(* Logix 5000 AddOnInstructionDefinition export Banner_Q5X_5000_Param_v4; software revision 33.00; part 3 of 3 *)
(* tags used below, declared in another part *)
   Q5X : Banner_Q5X_5000_v4;
   Port_Data : Banner_IOL_Port_v4;
   Port : DINT;
   Local_Control : DINT;
   Command_Being_Processed : BOOL;
   Update_Archive : BOOL;
   Index_Write_Inprocess : INT;
   Inprocess_Index : DINT;
(* Banner_Q5X_5000_Param_v4, continued *)

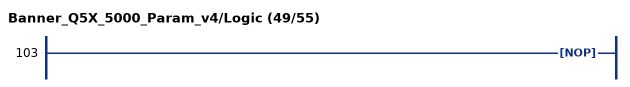
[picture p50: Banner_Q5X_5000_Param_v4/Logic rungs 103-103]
   103: NOP();
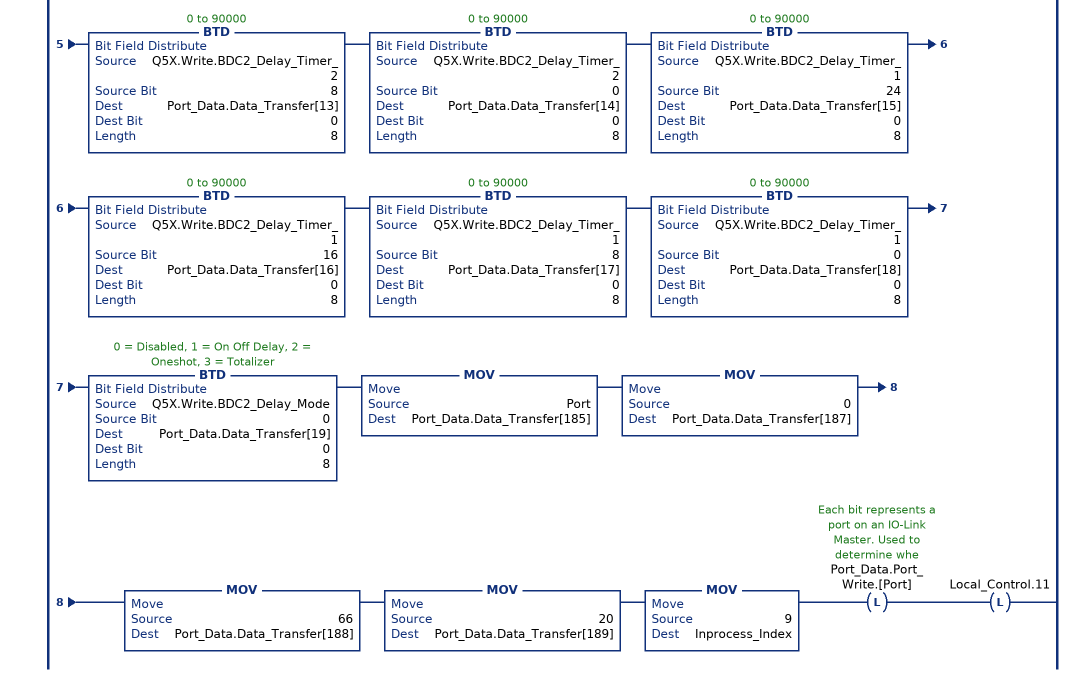
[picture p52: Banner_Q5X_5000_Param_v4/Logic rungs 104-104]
   // ************************************************************************************************************
   // Section of AOI that controls writing of the BDC2 Vendor Specific Configuration parameter (index 66).
   // ************************************************************************************************************
   104: XIC(Q5X.Initial_Global_Read)XIO(Command_Being_Processed)XIO(Local_Control.11)EQU(Q5X.Command,51)OTL(Command_Being_Processed)BTD(Q5X.Write.BDC2_Auto_Thresholding,0,Port_Data.Data_Transfer[0],0,8)BTD(Q5X.Write.BDC2_User_FGS_Window_Size,24,Port_Data.Data_Transfer[1],0,8)BTD(Q5X.Write.BDC2_User_FGS_Window_Size,16,Port_Data.Data_Transfer[2],0,8)BTD(Q5X.Write.BDC2_User_FGS_Window_Size,8,Port_Data.Data_Transfer[3],0,8)BTD(Q5X.Write.BDC2_User_FGS_Window_Size,0,Port_Data.Data_Transfer[4],0,8)BTD(Q5X.Write.BDC2_User_Teach_Offset,24,Port_Data.Data_Transfer[5],0,8)BTD(Q5X.Write.BDC2_User_Teach_Offset,16,Port_Data.Data_Transfer[6],0,8)BTD(Q5X.Write.BDC2_User_Teach_Offset,8,Port_Data.Data_Transfer[7],0,8)BTD(Q5X.Write.BDC2_User_Teach_Offset,0,Port_Data.Data_Transfer[8],0,8)BTD(Q5X.Write.BDC2_FGS_Window_Size,0,Port_Data.Data_Transfer[9],0,8)BTD(Q5X.Write.BDC2_BGS_Teach_Offset,0,Port_Data.Data_Transfer[10],0,8)BTD(Q5X.Write.BDC2_Delay_Timer_2,24,Port_Data.Data_Transfer[11],0,8)BTD(Q5X.Write.BDC2_Delay_Timer_2,16,Port_Data.Data_Transfer[12],0,8)BTD(Q5X.Write.BDC2_Delay_Timer_2,8,Port_Data.Data_Transfer[13],0,8)BTD(Q5X.Write.BDC2_Delay_Timer_2,0,Port_Data.Data_Transfer[14],0,8)BTD(Q5X.Write.BDC2_Delay_Timer_1,24,Port_Data.Data_Transfer[15],0,8)BTD(Q5X.Write.BDC2_Delay_Timer_1,16,Port_Data.Data_Transfer[16],0,8)BTD(Q5X.Write.BDC2_Delay_Timer_1,8,Port_Data.Data_Transfer[17],0,8)BTD(Q5X.Write.BDC2_Delay_Timer_1,0,Port_Data.Data_Transfer[18],0,8)BTD(Q5X.Write.BDC2_Delay_Mode,0,Port_Data.Data_Transfer[19],0,8)MOV(Port,Port_Data.Data_Transfer[185])MOV(0,Port_Data.Data_Transfer[187])MOV(66,Port_Data.Data_Transfer[188])MOV(20,Port_Data.Data_Transfer[189])MOV(9,Inprocess_Index)OTL(Port_Data.Port_Write.[Port])OTL(Local_Control.11);
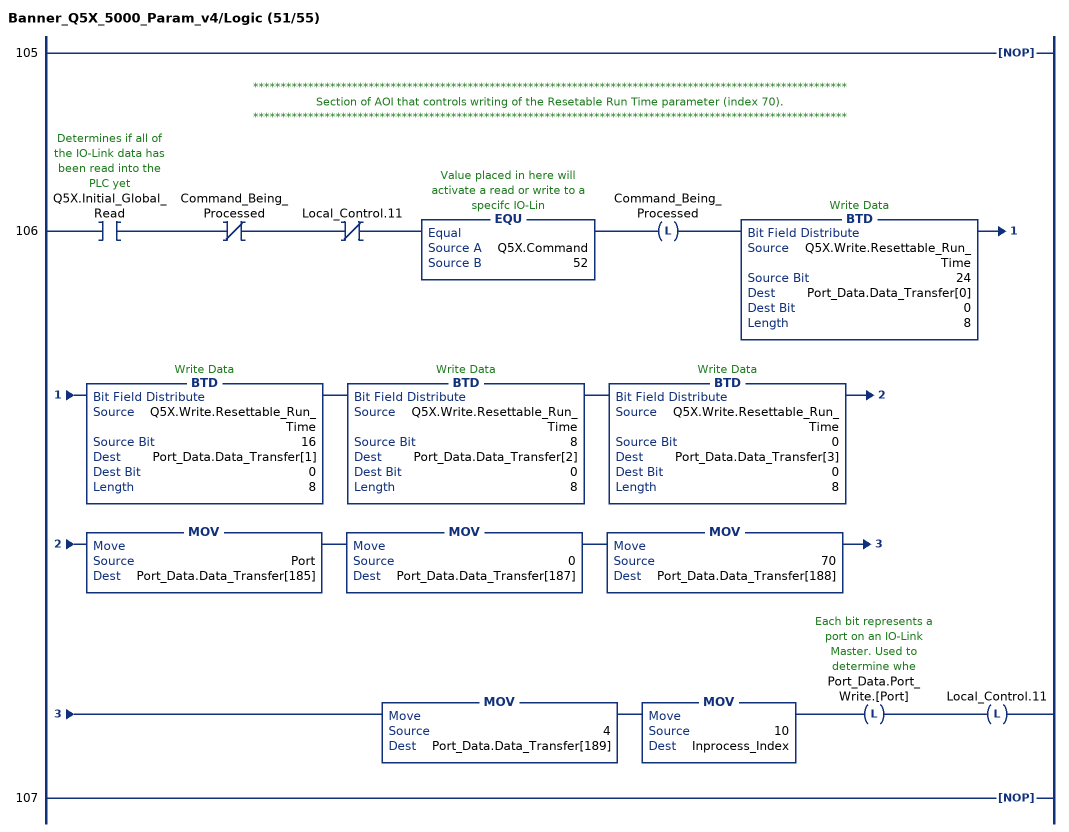
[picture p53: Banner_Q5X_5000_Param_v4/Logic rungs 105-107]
   105: NOP();
   // ************************************************************************************************************
   // Section of AOI that controls writing of the Resetable Run Time parameter (index 70).
   // ************************************************************************************************************
   106: XIC(Q5X.Initial_Global_Read)XIO(Command_Being_Processed)XIO(Local_Control.11)EQU(Q5X.Command,52)OTL(Command_Being_Processed)BTD(Q5X.Write.Resettable_Run_Time,24,Port_Data.Data_Transfer[0],0,8)BTD(Q5X.Write.Resettable_Run_Time,16,Port_Data.Data_Transfer[1],0,8)BTD(Q5X.Write.Resettable_Run_Time,8,Port_Data.Data_Transfer[2],0,8)BTD(Q5X.Write.Resettable_Run_Time,0,Port_Data.Data_Transfer[3],0,8)MOV(Port,Port_Data.Data_Transfer[185])MOV(0,Port_Data.Data_Transfer[187])MOV(70,Port_Data.Data_Transfer[188])MOV(4,Port_Data.Data_Transfer[189])MOV(10,Inprocess_Index)OTL(Port_Data.Port_Write.[Port])OTL(Local_Control.11);
   107: NOP();
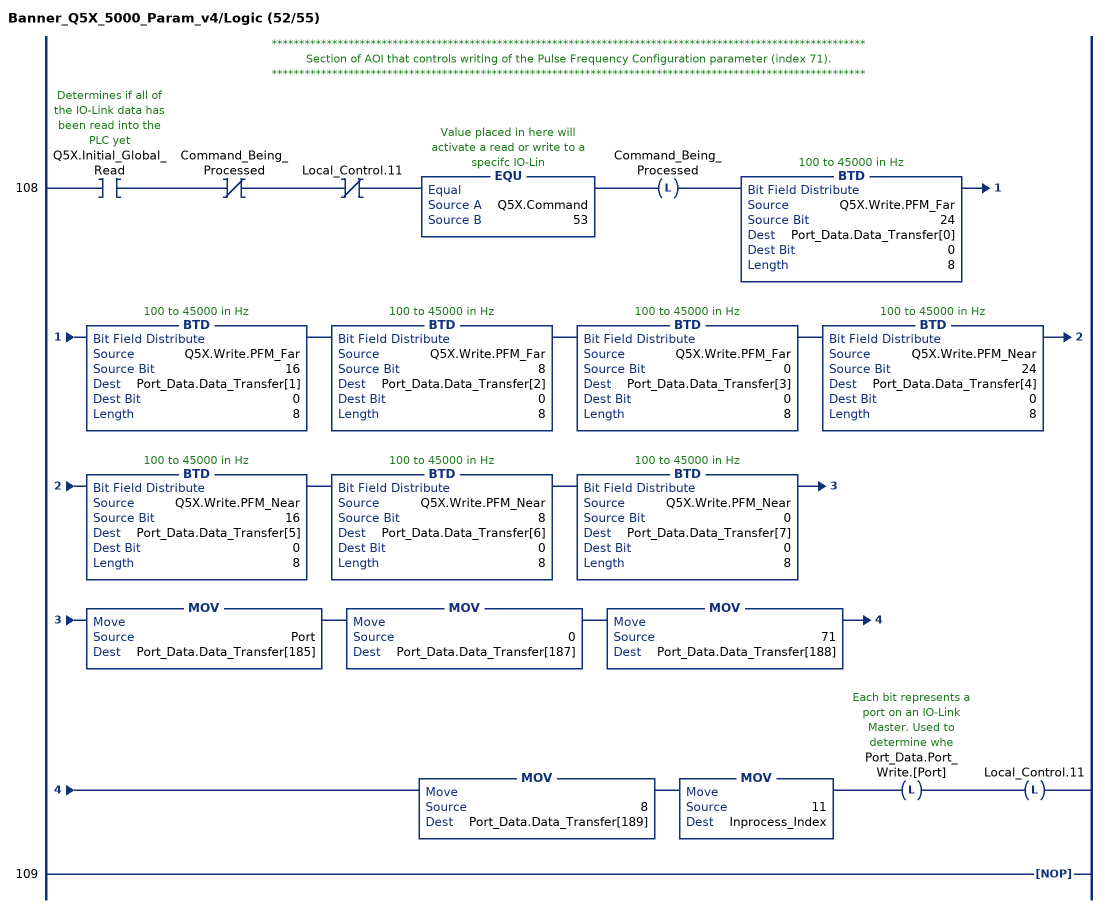
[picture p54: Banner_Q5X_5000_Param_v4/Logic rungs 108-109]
   // ************************************************************************************************************
   // Section of AOI that controls writing of the Pulse Frequency Configuration parameter (index 71).
   // ************************************************************************************************************
   108: XIC(Q5X.Initial_Global_Read)XIO(Command_Being_Processed)XIO(Local_Control.11)EQU(Q5X.Command,53)OTL(Command_Being_Processed)BTD(Q5X.Write.PFM_Far,24,Port_Data.Data_Transfer[0],0,8)BTD(Q5X.Write.PFM_Far,16,Port_Data.Data_Transfer[1],0,8)BTD(Q5X.Write.PFM_Far,8,Port_Data.Data_Transfer[2],0,8)BTD(Q5X.Write.PFM_Far,0,Port_Data.Data_Transfer[3],0,8)BTD(Q5X.Write.PFM_Near,24,Port_Data.Data_Transfer[4],0,8)BTD(Q5X.Write.PFM_Near,16,Port_Data.Data_Transfer[5],0,8)BTD(Q5X.Write.PFM_Near,8,Port_Data.Data_Transfer[6],0,8)BTD(Q5X.Write.PFM_Near,0,Port_Data.Data_Transfer[7],0,8)MOV(Port,Port_Data.Data_Transfer[185])MOV(0,Port_Data.Data_Transfer[187])MOV(71,Port_Data.Data_Transfer[188])MOV(8,Port_Data.Data_Transfer[189])MOV(11,Inprocess_Index)OTL(Port_Data.Port_Write.[Port])OTL(Local_Control.11);
   109: NOP();
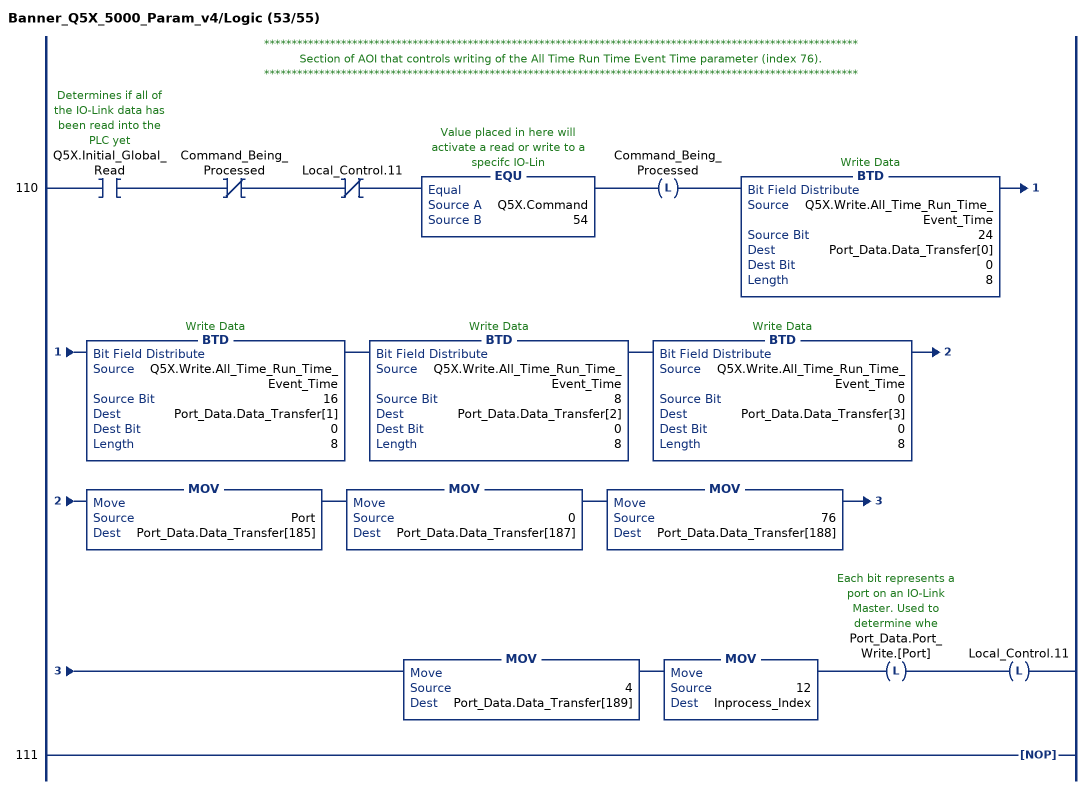
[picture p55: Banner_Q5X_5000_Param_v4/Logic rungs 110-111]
   // ************************************************************************************************************
   // Section of AOI that controls writing of the All Time Run Time Event Time parameter (index 76).
   // ************************************************************************************************************
   110: XIC(Q5X.Initial_Global_Read)XIO(Command_Being_Processed)XIO(Local_Control.11)EQU(Q5X.Command,54)OTL(Command_Being_Processed)BTD(Q5X.Write.All_Time_Run_Time_Event_Time,24,Port_Data.Data_Transfer[0],0,8)BTD(Q5X.Write.All_Time_Run_Time_Event_Time,16,Port_Data.Data_Transfer[1],0,8)BTD(Q5X.Write.All_Time_Run_Time_Event_Time,8,Port_Data.Data_Transfer[2],0,8)BTD(Q5X.Write.All_Time_Run_Time_Event_Time,0,Port_Data.Data_Transfer[3],0,8)MOV(Port,Port_Data.Data_Transfer[185])MOV(0,Port_Data.Data_Transfer[187])MOV(76,Port_Data.Data_Transfer[188])MOV(4,Port_Data.Data_Transfer[189])MOV(12,Inprocess_Index)OTL(Port_Data.Port_Write.[Port])OTL(Local_Control.11);
   111: NOP();
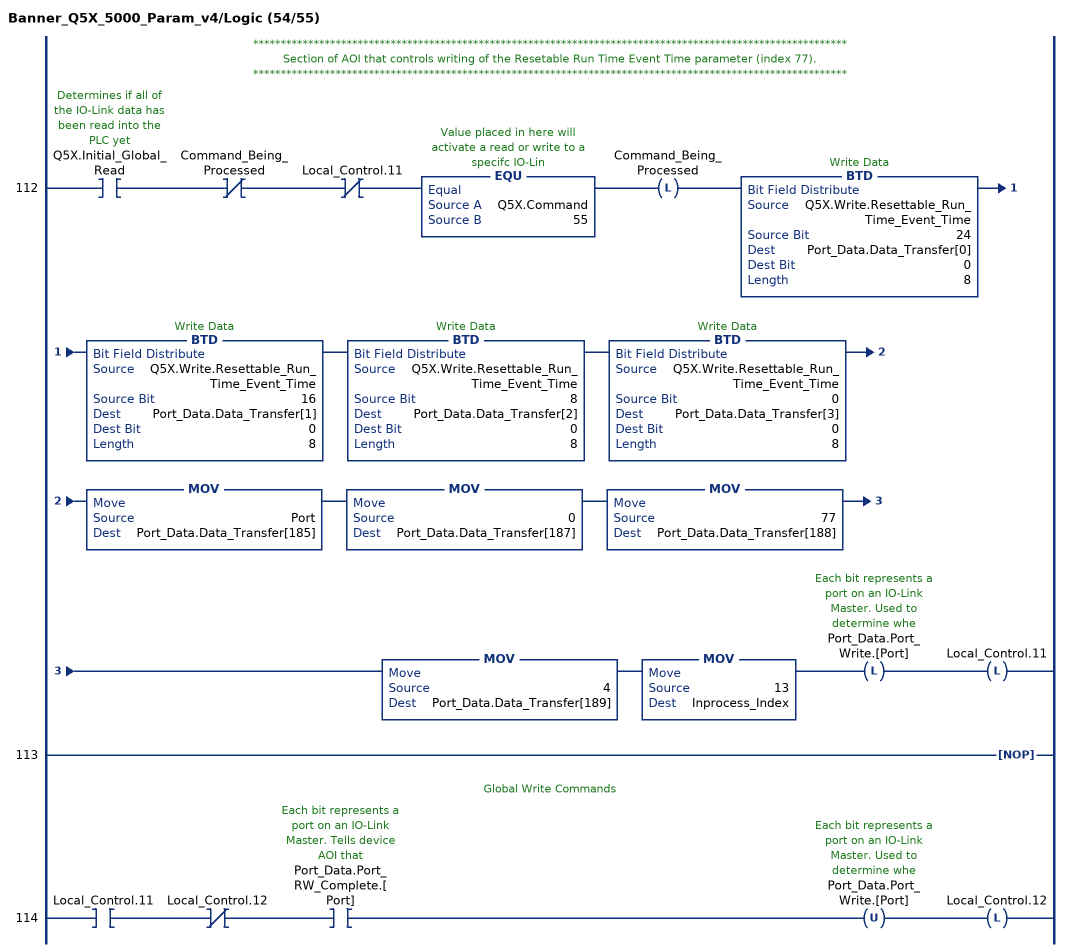
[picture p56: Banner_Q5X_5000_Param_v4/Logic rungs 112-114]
   // ************************************************************************************************************
   // Section of AOI that controls writing of the Resetable Run Time Event Time parameter (index 77).
   // ************************************************************************************************************
   112: XIC(Q5X.Initial_Global_Read)XIO(Command_Being_Processed)XIO(Local_Control.11)EQU(Q5X.Command,55)OTL(Command_Being_Processed)BTD(Q5X.Write.Resettable_Run_Time_Event_Time,24,Port_Data.Data_Transfer[0],0,8)BTD(Q5X.Write.Resettable_Run_Time_Event_Time,16,Port_Data.Data_Transfer[1],0,8)BTD(Q5X.Write.Resettable_Run_Time_Event_Time,8,Port_Data.Data_Transfer[2],0,8)BTD(Q5X.Write.Resettable_Run_Time_Event_Time,0,Port_Data.Data_Transfer[3],0,8)MOV(Port,Port_Data.Data_Transfer[185])MOV(0,Port_Data.Data_Transfer[187])MOV(77,Port_Data.Data_Transfer[188])MOV(4,Port_Data.Data_Transfer[189])MOV(13,Inprocess_Index)OTL(Port_Data.Port_Write.[Port])OTL(Local_Control.11);
   113: NOP();
   // Global Write Commands
   114: XIC(Local_Control.11)XIO(Local_Control.12)XIC(Port_Data.Port_RW_Complete.[Port])OTU(Port_Data.Port_Write.[Port])OTL(Local_Control.12);
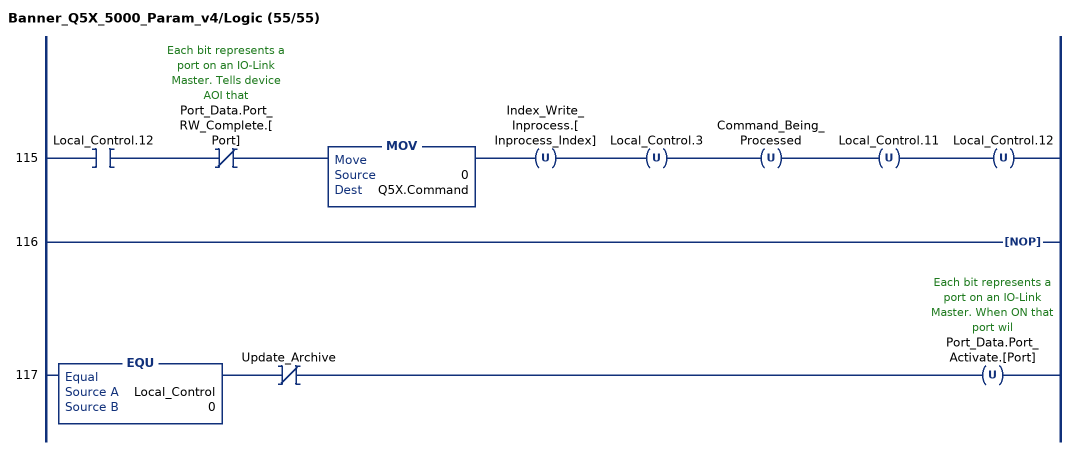
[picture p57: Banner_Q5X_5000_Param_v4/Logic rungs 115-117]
   115: XIC(Local_Control.12)XIO(Port_Data.Port_RW_Complete.[Port])MOV(0,Q5X.Command)OTU(Index_Write_Inprocess.[Inprocess_Index])OTU(Local_Control.3)OTU(Command_Being_Processed)OTU(Local_Control.11)OTU(Local_Control.12);
   116: NOP();
   117: EQU(Local_Control,0)XIO(Update_Archive)OTU(Port_Data.Port_Activate.[Port]);
END_ROUTINE
END_ADD_ON_INSTRUCTION
